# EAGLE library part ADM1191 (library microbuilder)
ADM1191 - I2C Digital Power Monitor 3.15V to 26V Operation 12-bit ADC Precision Current Sense Amplifier Precision Voltage Input Digikey: ADM1191-2ARMZ-R7TR-ND
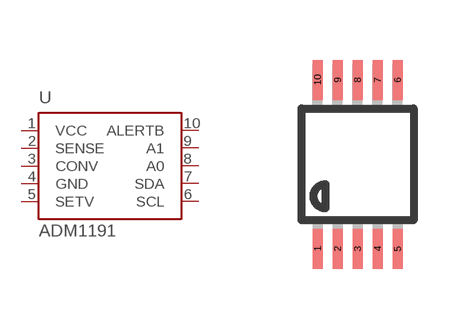
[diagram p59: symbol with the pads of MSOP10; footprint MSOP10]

Designator prefix U

## ADM1191  [MSOP10]
1  VCC
2  SENSE
3  CONV
4  GND
5  SETV
6  SCL
7  SDA
8  A0
9  A1
10  ALERTB

## Footprint MSOP10 (pad centres in mm)
10-Lead Mini Small Outline Package [MSOP]
smd 0.25 x 1: 1 -1,-2.113; 2 -0.5,-2.113; 3 0,-2.113; 4 0.5,-2.113; 5 1,-2.113; 6 1,2.113; 7 0.5,2.113; 8 0,2.113; 9 -0.5,2.113; 10 -1,2.113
